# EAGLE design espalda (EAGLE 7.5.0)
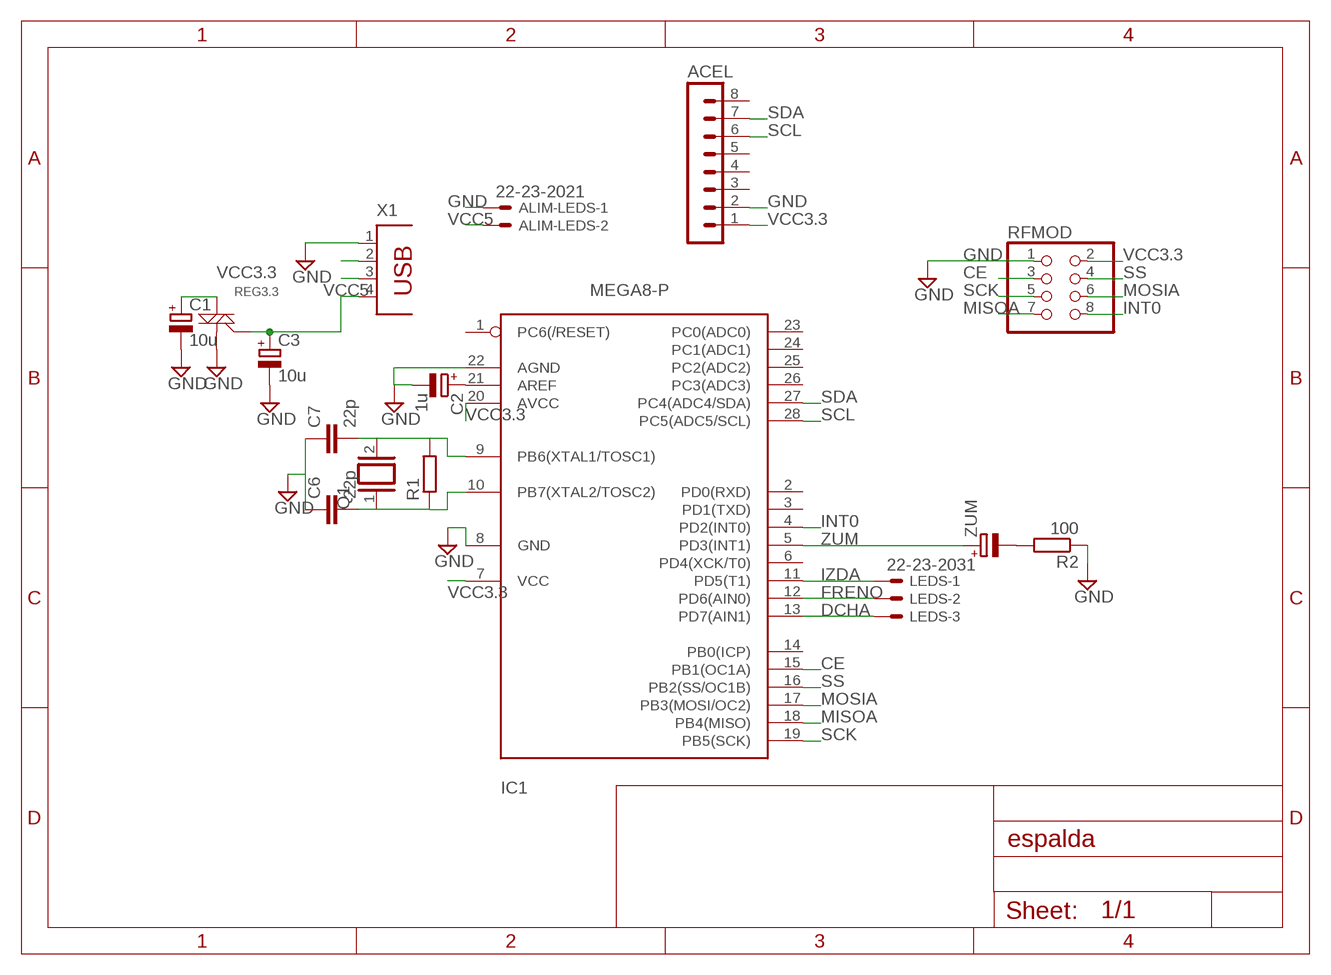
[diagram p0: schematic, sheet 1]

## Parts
ACEL  MA08-1  [MA08-1]
ALIM-LEDS  22-23-2021  [22-23-2021]
C1  10u  CPOL-EUE5-6  [E5-6]
C2  1u  CPOL-EUE5-6  [E5-6]
C3  10u  CPOL-EUE5-6  [E5-6]
C6  22p  C-EUC3216  [C3216]
C7  22p  C-EUC3216  [C3216]
IC1  MEGA8-P  [DIL28-3]
LEDS  22-23-2031  [22-23-2031]
Q1  XTAL/S  [QS]
R1  R-EU_0204/7  [0204/7]
R2  100  R-EU_0204/7  [0204/7]
REG3.3  TRIACSMD  [SOT223]
RFMOD  PINHD-2X4  [2X04]
X1  PN87520  [PN87520]
ZUM  CPOL-EUE5-13  [E5-13]

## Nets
CE: IC1.15(PB1(OC1A)) RFMOD.3
DCHA: IC1.13(PD7(AIN1)) LEDS.3
FRENO: IC1.12(PD6(AIN0)) LEDS.2
GND: ACEL.2 ALIM-LEDS.1 C1.- C2.- C3.- C6.1 C7.1 IC1.8(GND) IC1.22(AGND) R2.1 REG3.3.1(M1) RFMOD.1 X1.1
INT0: IC1.4(PD2(INT0)) RFMOD.8
IZDA: IC1.11(PD5(T1)) LEDS.1
MISOA: IC1.18(PB4(MISO)) RFMOD.7
MOSIA: IC1.17(PB3(MOSI/OC2)) RFMOD.6
N$1: C7.2 IC1.9(PB6(XTAL1/TOSC1)) Q1.2 R1.2
N$2: C6.2 IC1.10(PB7(XTAL2/TOSC2)) Q1.1 R1.1
N$3: C2.+ IC1.21(AREF)
N$6: R2.2 ZUM.-
N$7: X1.2
N$10: X1.3
SCK: IC1.19(PB5(SCK)) RFMOD.5
SCL: ACEL.6 IC1.28(PC5(ADC5/SCL))
SDA: ACEL.7 IC1.27(PC4(ADC4/SDA))
SS: IC1.16(PB2(SS/OC1B)) RFMOD.4
VCC3.3: ACEL.1 C1.+ IC1.7(VCC) IC1.20(AVCC) REG3.3.2(M2) RFMOD.2
VCC5: ALIM-LEDS.2 C3.+ REG3.3.3(G) X1.4
ZUM: IC1.5(PD3(INT1)) ZUM.+
Unconnected: ACEL.3 ACEL.4 ACEL.5 ACEL.8 IC1.1(PC6(/RESET)) IC1.2(PD0(RXD)) IC1.3(PD1(TXD)) IC1.6(PD4(XCK/T0)) IC1.14(PB0(ICP)) IC1.23(PC0(ADC0)) IC1.24(PC1(ADC1)) IC1.25(PC2(ADC2)) IC1.26(PC3(ADC3))

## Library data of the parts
ACEL = con-lstb:MA08-1: PIN HEADER; OC_FARNELL: unknown; OC_NEWARK: unknown
ALIM-LEDS = con-molex:22-23-2021: .100" (2.54mm) Center Header - 2 Pin; MF: MOLEX; MPN: 22-23-2021; OC_FARNELL: 1462926; OC_NEWARK: 25C3832
C1-C3 ZUM = resistor:CPOL-EU: POLARIZED CAPACITOR, European symbol
C6 C7 = resistor:C-EU: CAPACITOR, European symbol
IC1 = avr-6:MEGA8-P: MICROCONTROLLER 8 Kbytes FLASH 1 kbytes SRAM 512 bytes EEPROM USART 4-channel 10 bit ADC 2-channel 8 bit ADC
LEDS = con-molex:22-23-2031: .100" (2.54mm) Center Header - 3 Pin; MF: MOLEX; MPN: 22-23-2031; OC_FARNELL: 1462950; OC_NEWARK: 30C0862
Q1 = special:XTAL/S: CRYSTAL
R1 R2 = resistor:R-EU_: RESISTOR, European symbol
REG3.3 = sot:TRIAC: Low-power generic TRIAC packages
RFMOD = pinhead:PINHD-2X4: PIN HEADER
X1 = con-berg:PN87520: BERG USB connector; OC_FARNELL: unknown; OC_NEWARK: unknown

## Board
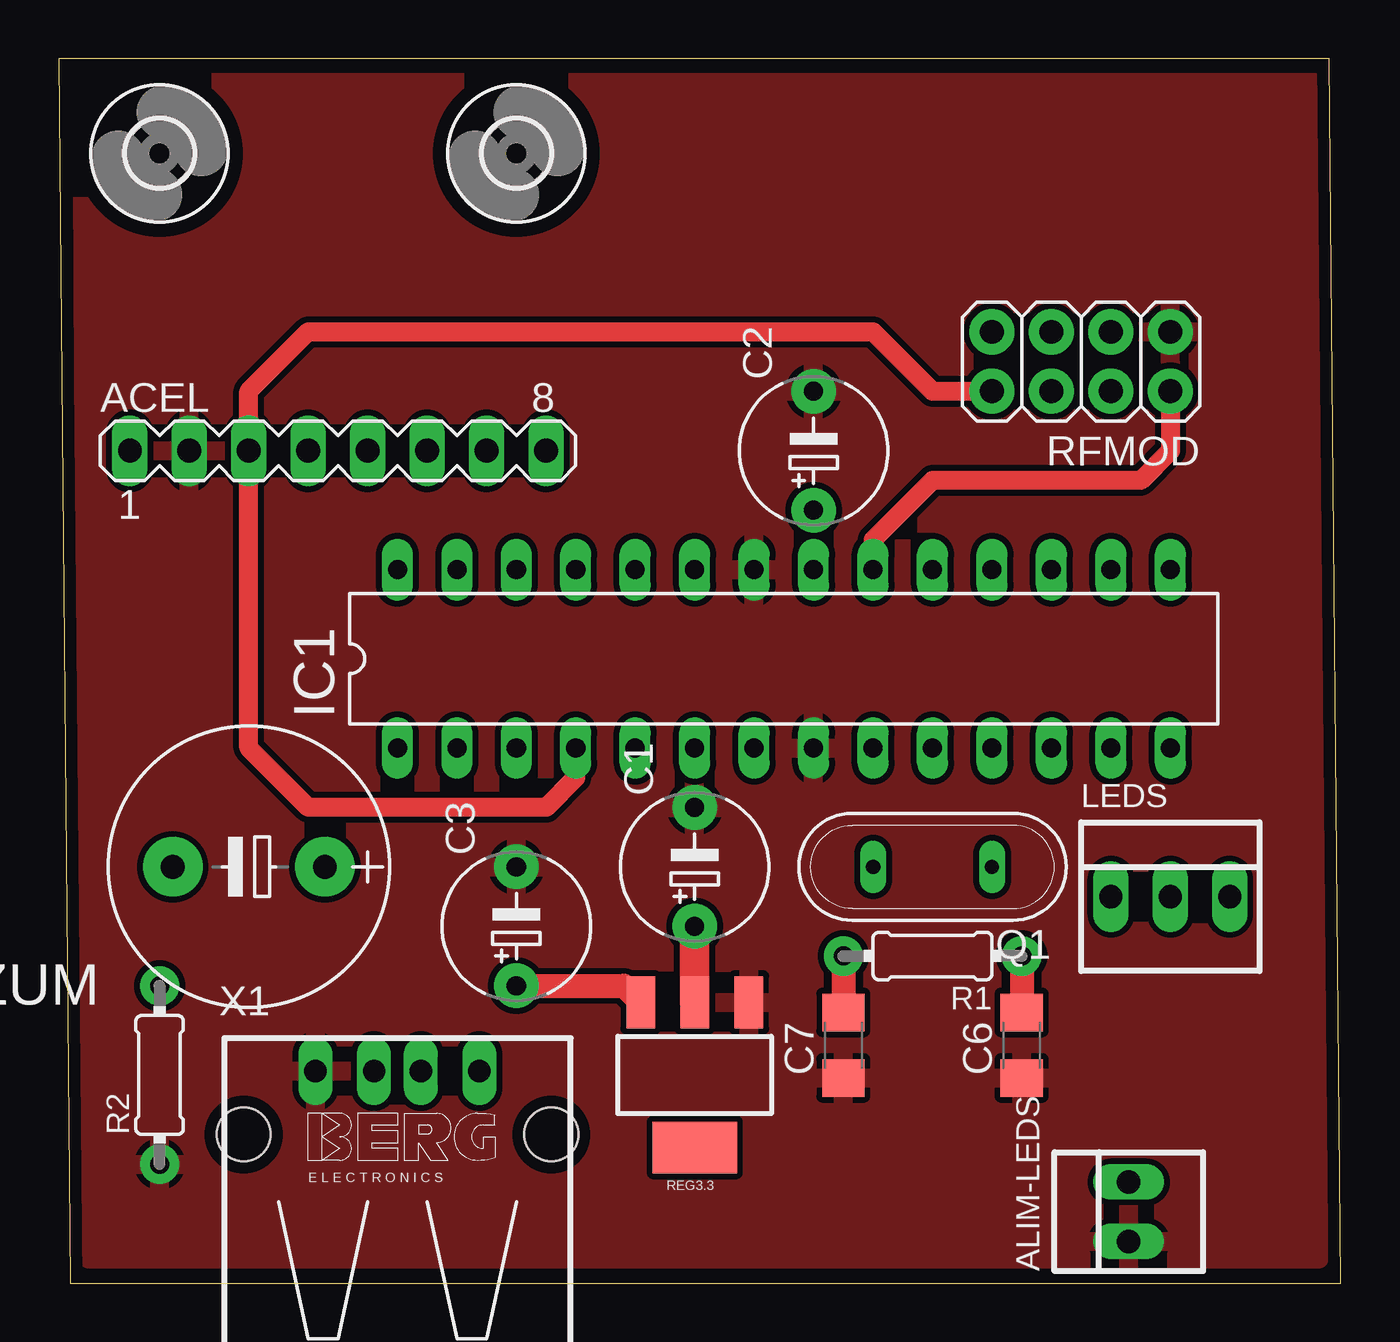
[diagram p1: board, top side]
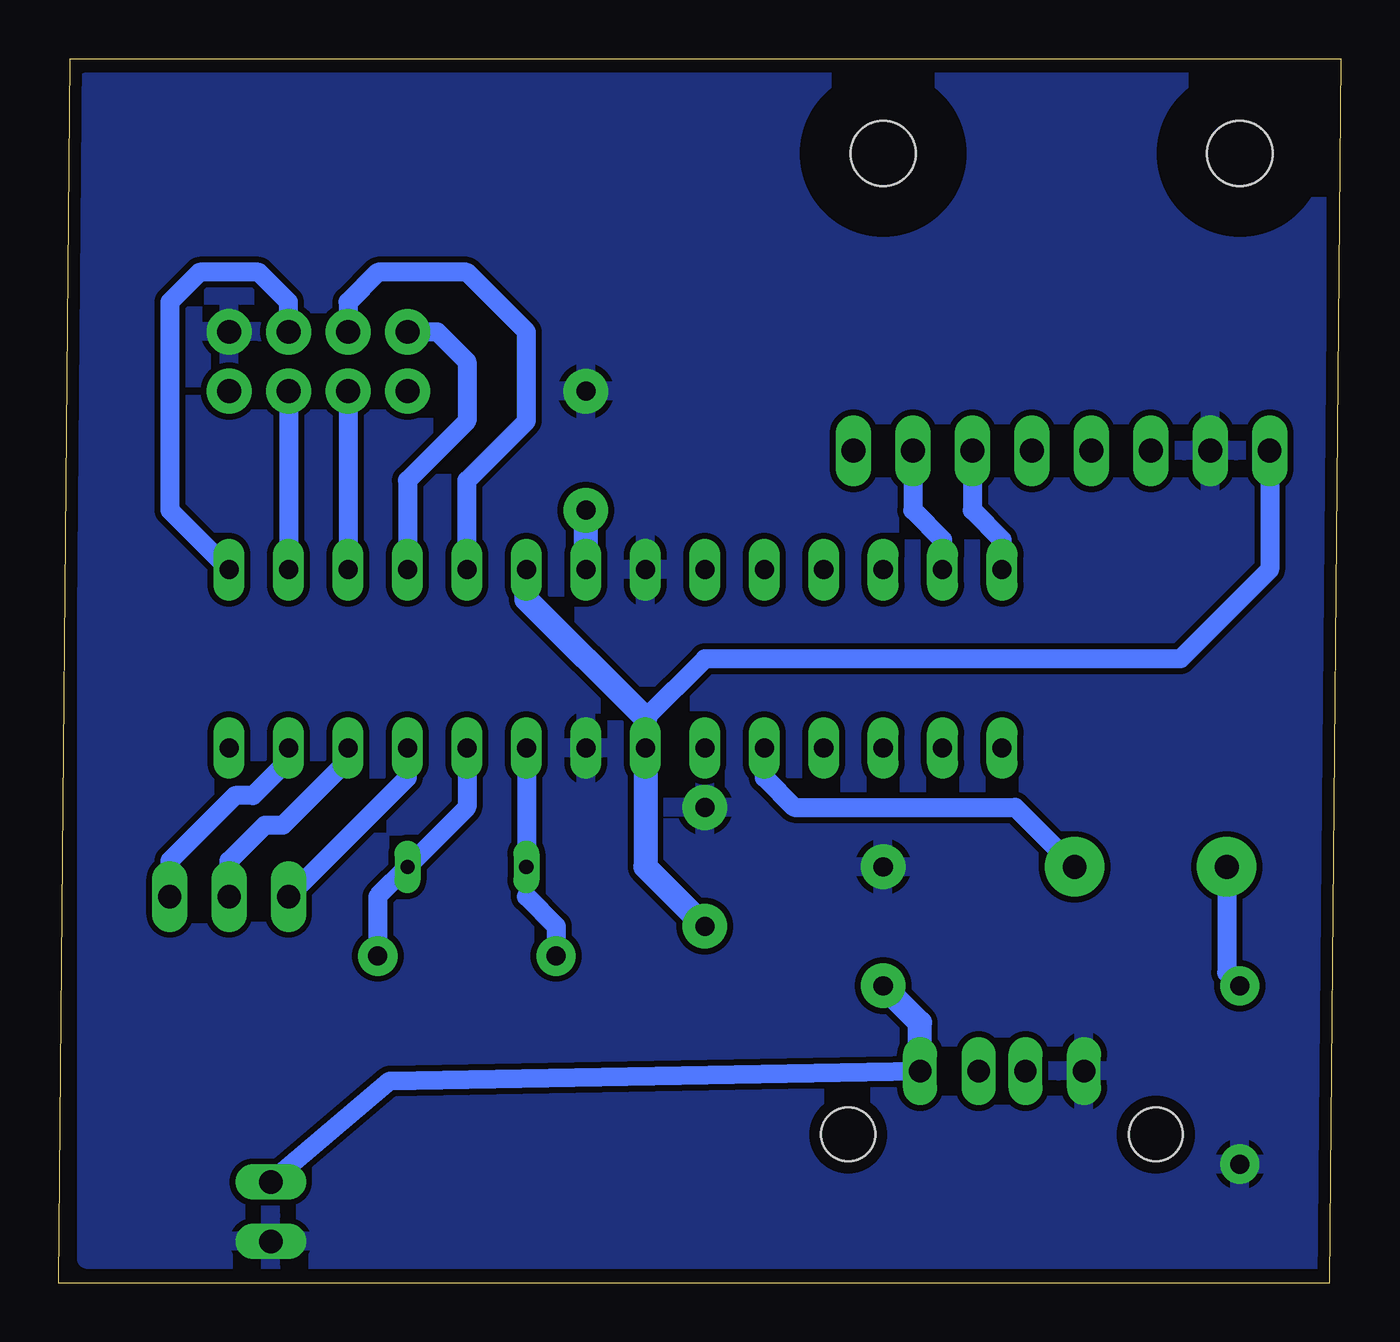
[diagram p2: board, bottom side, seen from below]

Size 54.79 x 52.31 mm. Coordinates in mm from the lower left corner, seen from the top.
Outline: 0.51,0 54.79,0 54.28,52.31 0,52.31 0.51,0
Copper layers (1*16): Top 0.035mm / dielectric 1.5mm / Bottom 0.035mm
Design rules "TE": minimum track width 12mil, minimum drill 23mil, track to track 10mil, track to pad 10mil, pad to pad 10mil, via to via 10mil, smd to smd 10mil, copper to edge 20mil, drill to drill 8mil, minimum pad ring 10mil, minimum via ring 8mil, stop-mask expansion 4mil, vias tented up to drill 0mil, thermal gap 10mil

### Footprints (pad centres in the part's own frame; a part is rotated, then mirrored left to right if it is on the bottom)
MA08-1 = drill 1.016 long: 1 -8.89,0; 2 -6.35,0; 3 -3.81,0; 4 -1.27,0; 5 1.27,0; 6 3.81,0; 7 6.35,0; 8 8.89,0
22-23-2021 = drill 1 long: 1 -1.27,0; 2 1.27,0
E5-6 = drill 0.813 pad 1.905: + -2.54,0; - 2.54,0
C3216 = smd 1.6 x 1.8: 1 -1.4,0; 2 1.4,0
DIL28-3 = drill 0.813 long: 1 -16.51,-3.81; 2 -13.97,-3.81; 3 -11.43,-3.81; 4 -8.89,-3.81; 5 -6.35,-3.81; 6 -3.81,-3.81; 7 -1.27,-3.81; 8 1.27,-3.81; 9 3.81,-3.81; 10 6.35,-3.81; 11 8.89,-3.81; 12 11.43,-3.81; 13 13.97,-3.81; 14 16.51,-3.81; 15 16.51,3.81; 16 13.97,3.81; 17 11.43,3.81; 18 8.89,3.81; 19 6.35,3.81; 20 3.81,3.81; 21 1.27,3.81; 22 -1.27,3.81; 23 -3.81,3.81; 24 -6.35,3.81; 25 -8.89,3.81; 26 -11.43,3.81; 27 -13.97,3.81; 28 -16.51,3.81
22-23-2031 = drill 1 long: 1 -2.54,0; 2 0,0; 3 2.54,0
QS = drill 0.61 long: 1 -2.54,0; 2 2.54,0
0204/7 = drill 0.813 pad 1.676: 1 -3.81,0; 2 3.81,0
SOT223 = smd 1.219 x 2.235: 1 -2.311,-3.099; 2 0,-3.099; 3 2.311,-3.099 | smd 3.6 x 2.2: 4 0,3.099
2X04 = drill 1.016 pad 1.93: 1 -3.81,-1.27; 2 -3.81,1.27; 3 -1.27,-1.27; 4 -1.27,1.27; 5 1.27,-1.27; 6 1.27,1.27; 7 3.81,-1.27; 8 3.81,1.27
2,8 = hole 2.8: 0,0
PN87520 = drill 0.95 long: 1 -3.5,2.71; 2 -1,2.71; 3 1,2.71; 4 3.5,2.71 | hole 2.3: -6.57,0; 6.57,0
E5-13 = drill 1.016 pad 2.54: + -3.25,0; - 3.25,0

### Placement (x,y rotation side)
ACEL  11.94,35.56 0 top
ALIM-LEDS  45.72,3.05 90 top
C1  27.18,17.78 90 top
C2  32.26,35.56 90 top
C3  19.56,15.24 90 top
C6  41.15,10.16 90 top
C7  33.53,10.16 90 top
IC1  30.99,26.67 0 top
LEDS  47.5,16.51 0 top
Q1  37.34,17.78 180 top
R1  37.34,13.97 180 top
R2  4.32,8.89 90 top
REG3.3  27.18,8.89 180 top
RFMOD  43.69,39.37 180 top
U$1  [2,8]  4.32,48.26 0 top
U$2  [2,8]  19.56,48.26 0 top
X1  14.48,6.35 0 top
ZUM  8.13,17.78 180 top

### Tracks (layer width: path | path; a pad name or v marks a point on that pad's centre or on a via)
CE
  Bottom 0.813: RFMOD.3 44.96,41.91 46.23,43.18 48.77,43.18 50.04,41.91 50.04,33.02 IC1.15
DCHA
  Bottom 0.813: IC1.13 44.96,22.35 46.48,20.83 47.24,20.83 50.04,18.03 LEDS.3
FRENO
  Bottom 0.813: IC1.12 42.42,22.35 45.21,19.56 45.97,19.56 47.5,18.03 LEDS.2
GND
  pour Bottom: 1.02,51.31 53.59,51.31 53.59,1.02 1.02,1.02
  pour Top: 1.02,51.31 53.59,51.31 53.85,1.02 1.27,1.02
INT0
  Top 0.813: IC1.4 22.1,21.59 20.83,20.32 10.67,20.32 8.13,22.86 8.13,38.1 10.67,40.64 34.8,40.64 37.34,38.1 RFMOD.8
IZDA
  Bottom 0.406: 39.88,21.59 39.88,22.1
  Bottom 0.813: IC1.11 39.88,22.1 | LEDS.1 39.88,21.59
MISOA
  Bottom 0.813: RFMOD.7 38.61,40.64 37.34,39.37 37.34,36.83 39.88,34.29 IC1.18
MOSIA
  Bottom 0.813: RFMOD.6 IC1.17
N$1
  Top 1.016: R1.2 C7.2
  Bottom 0.406: Q1.2 34.8,16.51
  Bottom 0.813: IC1.9 Q1.2 | 34.8,16.51 33.53,15.24 R1.2
N$2
  Top 1.016: R1.1 C6.2
  Bottom 0.813: IC1.10 37.34,20.32 Q1.1 41.15,16.51 R1.1
N$3
  Bottom 1.016: IC1.21 C2.+
N$6
  Bottom 0.813: ZUM.- 4.88,13.26 R2.2
SCK
  Bottom 0.813: IC1.19 37.34,34.29 34.8,36.83 34.8,40.64 37.34,43.18 41.15,43.18 42.42,41.91 RFMOD.5
SCL
  Bottom 0.813: ACEL.6 15.75,33.02 14.48,31.75 IC1.28
SDA
  Bottom 0.813: ACEL.7 18.29,33.02 17.02,31.75 IC1.27
SS
  Bottom 0.813: RFMOD.4 IC1.16
VCC3.3
  Top 0.813: RFMOD.2 47.5,35.56 46.23,34.29 37.34,34.29 34.8,31.75 IC1.20
  Top 1.27: C1.+ REG3.3.2
  Bottom 0.813: IC1.7 29.72,24.13 27.18,26.67 6.86,26.67 3.05,30.48 ACEL.1
  Bottom 1.016: 29.72,24.13 34.8,29.21 IC1.20 | IC1.7 29.72,17.78 C1.+
VCC5
  Top 1.016: C3.+ 24.15,12.7 REG3.3.3
  Bottom 0.813: ALIM-LEDS.2 40.64,8.64 X1.4
  Bottom 1.016: X1.4 17.98,11.12 C3.+
ZUM
  Bottom 0.813: IC1.5 24.64,21.59 23.37,20.32 13.92,20.32 ZUM.+

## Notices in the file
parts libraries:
sot: Licensing: Creative Commons ShareAlike 4.0 International - https://creativecommons.org/licenses/by-sa/4.0
